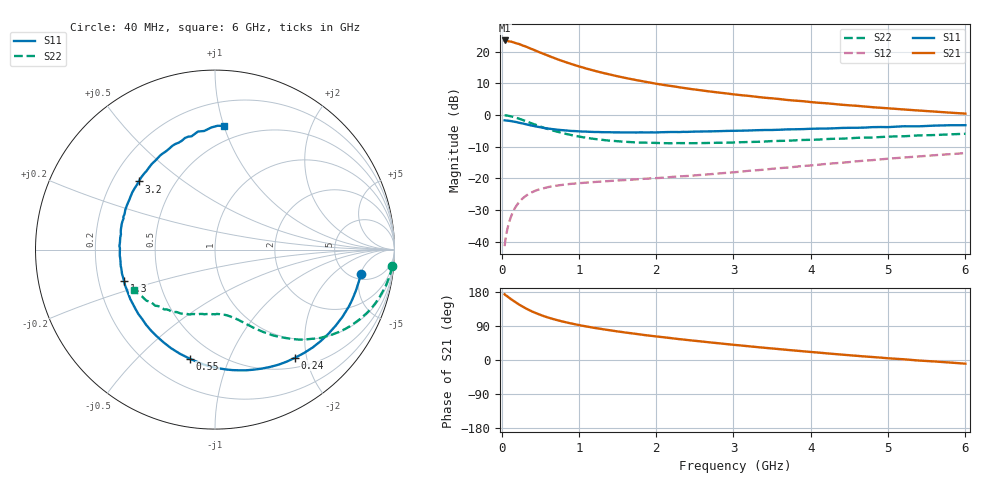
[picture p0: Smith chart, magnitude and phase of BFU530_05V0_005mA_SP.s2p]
! Filename:  P:\Prog\Test\Noise\ATS_data\Testdata_Net\03 Spar\BFU530_APG2013_40_A05_05p0V_005mA_SP_CM01_D.s2p
! Date/Time: Fri 26/Apr/2013 13:03:15
! BFU530_APG2013_40_A05_05p0V_1to25mA_SP_CM01_Bias4_R.s2p
! MDIF S-parameter v. bias file
! BFU530_APG2013_40_A05_05p0V_1to25mA_SP_CM01
! Date/time Wed Apr 24 19:36:53 2013
! VAR V_out= 5.0000
! VAR I_out= 4.9950
! VAR V_in= 0.8187
! VAR I_in= 0.0542
! Device data file deembeded for feedlines and parallel
! Original file: \03 Spar\BFU530_APG2013_40_A05_05p0V_005mA_SP_CM01_R.s2p
! Feed-files: PR047V01_250413_Feed1.s2p, PR047V01_250413_Feed2.s2p
! Parallel-file: PR047V01_250413_Par.s2p
# MHz S MA R 50
!  Freq-MHz  S11-mag  S11-arg  S21-mag  S21-arg  S12-mag  S12-arg  S22-mag  S22-arg
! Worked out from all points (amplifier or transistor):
!   98 points, 40 MHz to 6 GHz, reference 50 ohm
!   highest |S21| = 23.6 dB at 40 MHz (marker M1)
!   |S21| within 3 dB of that: start of sweep to 420.1 MHz
!   unconditionally stable (mu >= 1): 2.253 GHz to 4.416 GHz
!   at 300 MHz: K = 0.19, MSG = 23.8 dB, |S12| = -25.8 dB
!   at 1.6 GHz: K = 0.83, MSG = 16.1 dB, |S12| = -20.6 dB
!   at 6 GHz: K = 0.85, MSG = 6.2 dB, |S12| = -12.0 dB
!   S11 on the Smith chart (normalised r, x): 40 MHz: 6.01, -5.12; 240 MHz: 0.65, -1.80; 550 MHz: 0.37, -0.73; 1.3 GHz: 0.31, -0.15; 3.2 GHz: 0.31, +0.35; 6 GHz: 0.38, +1.00
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40  0.8252 -9.5  15.1 173.4  0.008458 84.4  0.9901 -5.4
50  0.8219 -11.8  15.1 171.2  0.01051 83.5  0.9894 -6.7
60  0.8195 -13.9  14.87 170.2  0.0126 82.4  0.9852 -8.2
140  0.7945 -32.4  14.28 158.1  0.028 72.8  0.9426 -18.4
240  0.7497 -53.5  13.07 144.8  0.04377 62.6  0.865 -29.6
320  0.7125 -68.5  12.03 135.6  0.05334 56.1  0.7971 -36.9
360  0.695 -75.4  11.46 131.6  0.05729 53.3  0.7647 -40.1
460  0.6551 -90.7  10.2 122.5  0.06511 47.7  0.6893 -46.7
550  0.6243 -102.9  9.21 115.5  0.06983 43.7  0.6279 -51.6
650  0.6013 -114.1  8.239 109.2  0.0745 40.6  0.5771 -56.0
750  0.5818 -123.9  7.415 103.6  0.07774 38.3  0.5338 -59.5
900  0.5605 -136.4  6.426 96.4  0.08169 36.0  0.4838 -63.9
1050  0.5484 -146.9  5.648 90.2  0.08459 34.6  0.4463 -67.6
1300  0.5359 -160.9  4.678 81.6  0.08901 33.6  0.4056 -72.7
1600  0.5303 -174.8  3.863 72.6  0.09381 33.7  0.3778 -78.2
2050  0.5343 169.4  3.055 61.1  0.1015 35.2  0.3606 -86.1
2450  0.5451 156.8  2.577 51.7  0.1096 36.7  0.3587 -93.5
3100  0.5658 140.0  2.061 38.2  0.1276 39.2  0.3719 -104.5
3200  0.5699 138.2  2.007 36.2  0.1314 39.5  0.3748 -105.9
4100  0.6101 118.2  1.565 19.5  0.1638 39.3  0.4091 -121.8
5200  0.6645 98.2  1.226 2.0  0.213 34.8  0.4616 -140.6
6000  0.691 85.8  1.053 -9.7  0.2501 29.1  0.5058 -153.8
